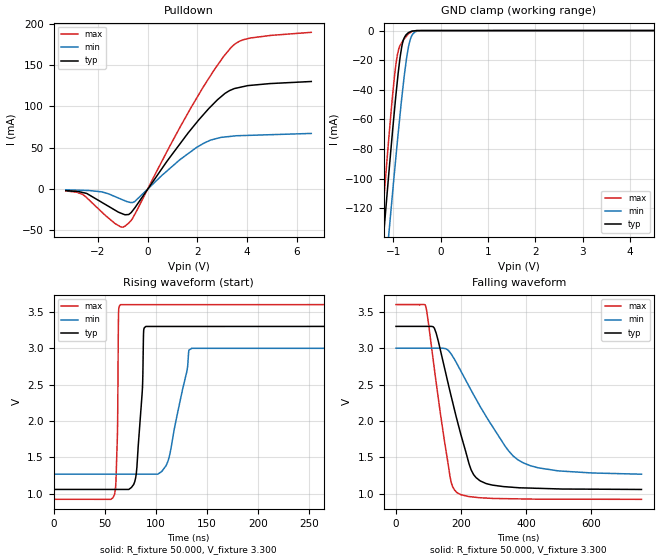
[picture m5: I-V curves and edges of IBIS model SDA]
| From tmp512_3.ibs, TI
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|   SDA   3.3V digital I/O_open_drain
[Model] SDA
Model_type I/O_open_drain
Polarity   Non-Inverting
Enable   Active-Low
Vinl = 0.8
Vinh = 2.1
Vmeas = 1.55
Vref = 1.55
Cref = 15pF
Rref = 50
|   typ   min   max
|   average of high and low output
C_comp   2.2160048E-11   1.8819970E-11   2.9413280E-11
|   output high - high impedance
|C_comp   2.5439350e-12   2.1052890e-12   3.0102690e-12
|   output low
|C_comp   4.1776160e-11   3.5534650e-11   5.5816290e-11
[Voltage Range]   3.3   3   3.6
[Temperature Range]   27   125   -40
[GND Clamp Reference]   0   0   0
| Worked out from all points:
|   slope of the pulldown table from 0 to 0.495 V, typ, clamps not added: 22.9 ohm
|   GND clamp passes 1 mA (typ) near -0.65 V on its own axis
|   falling waveform, R_fixture 50.000, V_fixture 3.300: 20-80 % time 75.8ns typ, 139ns min, 50.6ns max; typ from 3.3 V to 1.06 V
|   rising waveform, R_fixture 50.000, V_fixture 3.300: 20-80 % time 5.43ns typ, 15.2ns min, 1.59ns max; typ from 1.06 V to 3.3 V
[Pulldown]
|   Voltage   I(typ)   I(min)   I(max)
-3.3V     -1.937mA   -1.001mA   -2.312mA
-2.625V   -4.219mA   -1.614mA   -6.475mA
-1.328V   -25.43mA   -9.067mA   -41.55mA
-927mV    -31.1mA    -14.14mA   -45.17mA
-759.5mV  -30.76mA   -15.84mA   -41.07mA
-519.2mV  -22.81mA   -15.09mA   -30.59mA
862mV     37.03mA    24.07mA    50.32mA
1.973V    80.54mA    50.36mA    110.1mA
2.81V     108mA      61.33mA    149.8mA
3.355V    119.8mA    63.74mA    171.2mA
4.143V    125.4mA    64.97mA    182.8mA
6.59V     130.1mA    67.24mA    189.6mA
[GND Clamp]
|   Voltage   I(typ)   I(min)   I(max)
-3.3V     -991.7mA   -982.8mA   -1.027A
-1.273V   -165.8mA   -203.5mA   -145.3mA
-1.227V   -147.9mA   -186.4mA   -126.1mA
-1.181V   -130.2mA   -169.8mA   -107.6mA
-1.084V   -93.62mA   -134.8mA   -69.48mA
-935.4mV  -41.35mA   -82.99mA   -21.15mA
-880mV    -24.83mA   -64.76mA   -12.13mA
-821.8mV  -11.41mA   -46.33mA   -8.323mA
-716.8mV  -2.556mA   -18.5mA    -3.668mA
-608.1mV  -407uA     -3.59mA    -733.3uA
-400.2mV  -35.95uA   -27.99uA   -50.57uA
6.59V     0A         0A         0A
[POWER Clamp]
|   SCR cell for ESD function. Effects occurr above VDD x 2
|   Voltage   I(typ)   I(min)   I(max)
-3.3V     0A         0A         0A
0V        0A         0A         0A
6.6V      0A         0A         0A
[Ramp]
R_load = 50
|   typ   min   max
dV/dt_r   1.3275/5.41366e-009   1.01803/1.51838e-008   1.5872/1.58446e-009
dV/dt_f   1.32699/7.56536e-008   1.0114/1.3816e-007   1.58717/5.05622e-008
[Falling Waveform]
R_fixture = 50.000
V_fixture = 3.300
V_fixture_min = 3.000
V_fixture_max = 3.600
C_fixture = 0.000
|  time   V(typ)   V(min)   V(max)
0s        3.301V     3.001V     3.601V
91.31ns   3.301V     3.001V     3.578V
118.4ns   3.27V      3.001V     2.696V
166ns     2.403V     2.941V     1.232V
187.3ns   2.015V     2.785V     1.014V
225ns     1.4V       2.47V      959.2mV
245.6ns   1.221V     2.301V     948.6mV
377.2ns   1.08V      1.458V     927.5mV
498.6ns   1.065V     1.313V     923.1mV
753.7ns   1.057V     1.267V     921.3mV
[Rising Waveform]
R_fixture = 50.000
V_fixture = 3.300
V_fixture_min = 3.000
V_fixture_max = 3.600
C_fixture = 0.000
|  time   V(typ)   V(min)   V(max)
0s        1.057V     1.267V     921.3mV
59.63ns   1.057V     1.267V     985.7mV
62.49ns   1.057V     1.267V     1.807V
63.65ns   1.057V     1.267V     3.509V
65.49ns   1.057V     1.267V     3.599V
80.34ns   1.218V     1.267V     3.599V
90.33ns   3.299V     1.267V     3.599V
111.9ns   3.299V     1.445V     3.599V
135.1ns   3.299V     2.998V     3.599V
753.7ns   3.301V     3.001V     3.601V
